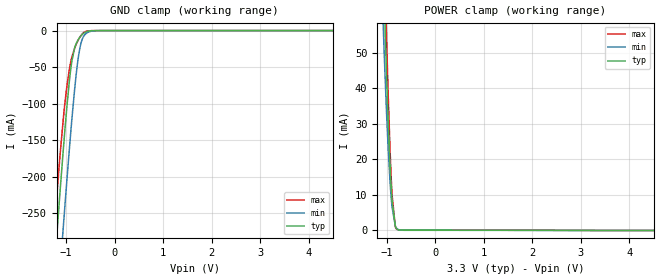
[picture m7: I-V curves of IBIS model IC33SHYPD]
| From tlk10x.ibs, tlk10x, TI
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|   Model
[Model]   IC33SHYPD
Model_type   Input
Vinl = 0.99
Vinh = 2.31
|   typ   min   max
C_comp   1.472pF   1.437pF   1.515pF
[Voltage Range]   3.3   3   3.6
[Temperature Range]   25   125   -40
[Power Clamp Reference]   3.3   3   3.6
[GND Clamp Reference]   -0   -0   -0
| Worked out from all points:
|   GND clamp passes 1 mA (typ) near -0.56 V on its own axis
|   POWER clamp passes 1 mA (typ) near -0.82 V on its own axis
[GND Clamp]
|   Voltage   I(typ)   I(min)   I(max)
-3.3V     -2.326A    -2.431A    -2.267A
-1.251V   -331.2mA   -441.1mA   -274.2mA
-1.142V   -233mA     -341.3mA   -181.8mA
-1.063V   -164.7mA   -270.5mA   -122.4mA
-983.4mV  -102mA     -201.9mA   -74.68mA
-884.4mV  -41.82mA   -121.8mA   -36.2mA
-825mV    -23.18mA   -79.07mA   -23.87mA
-745.8mV  -11.7mA    -34.44mA   -12.15mA
-686.4mV  -6.491mA   -15.06mA   -5.887mA
-607.2mV  -2.286mA   -4.91mA    -1.487mA
-270.6mV  -12.2uA    -24.65uA   -14.76uA
6.59V     0A         0A         0A
[POWER Clamp]
|   Voltage   I(typ)   I(min)   I(max)
-3.3V     1.527A     1.443A     1.596A
-1.082V   79.36mA    60.6mA     96.26mA
-1.063V   69.47mA    52.83mA    84.84mA
-1.053V   64.69mA    49.1mA     79.25mA
-1.013V   46.83mA    35.26mA    57.91mA
-1.003V   42.71mA    32.08mA    52.89mA
-973.5mV  31.25mA    23.3mA     38.77mA
-933.9mV  18.27mA    13.58mA    22.6mA
-894.3mV  8.564mA    6.666mA    10.23mA
-825mV    1.124mA    1.267mA    957.6uA
-785.4mV  329.4uA    448.3uA    292.2uA
6.59V     0A         0A         0A
